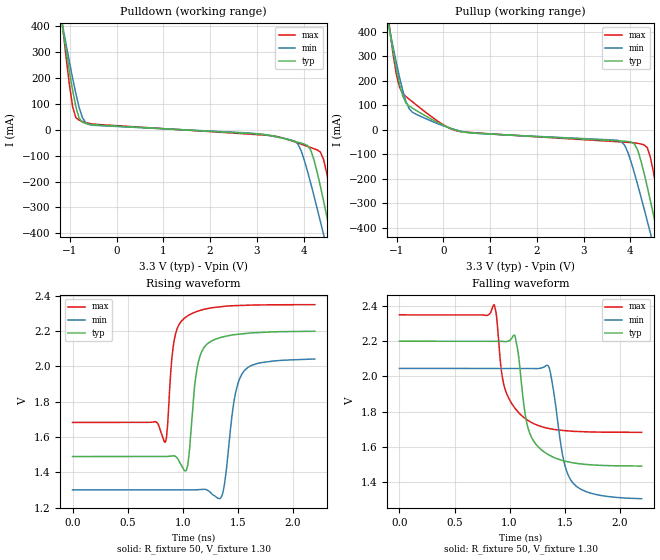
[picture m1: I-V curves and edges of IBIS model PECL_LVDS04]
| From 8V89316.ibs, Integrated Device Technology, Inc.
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[Model]   PECL_LVDS04
|LVPECL Driver
Model_type   Output_ECL
Polarity   Non-Inverting
|   typ   min   max
C_comp   2pF   1.5pF   2.5pF
Vmeas = 1.95V
Rref = 50
Cref = 0
Vref = 1.3V
|   typ   min   max
[Voltage range]   3.3V   3.135V   3.465V
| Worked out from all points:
|   rising waveform, R_fixture 50, V_fixture 1.30: 20-80 % time 82.3ps typ, 95.1ps min, 74.8ps max; typ from 1.49 V to 2.2 V
|   falling waveform, R_fixture 50, V_fixture 1.30: 20-80 % time 127ps typ, 118ps min, 154ps max; typ from 2.2 V to 1.49 V
[Pulldown]
|Voltage   I (typ)   I (min)   I (max)
-3.3V     3.045A     2.601A     4.065A
-1.146V   383.9mA    395mA      387.6mA
-939.2mV  152.8mA    199.5mA    89.52mA
-801.5mV  45.92mA    87.39mA    37.53mA
-594.9mV  22.04mA    20.74mA    25.14mA
3.811V    -44.66mA   -43.56mA   -46.44mA
3.949V    -51.54mA   -81mA      -55.19mA
4.156V    -79.05mA   -207.7mA   -68.56mA
4.431V    -276.5mA   -406.1mA   -115.7mA
4.51V     -344.5mA   -464.8mA   -180.2mA
4.928V    -719.3mA   -781.2mA   -653.8mA
6.6V      -2.246A    -2.062A    -2.647A
[Pullup]
|Voltage   I (typ)   I (min)   I (max)
-3.3V     3.045A     2.599A     4.069A
-1.215V   477.4mA    471.2mA    517.2mA
-1.146V   397.5mA    404.2mA    408.4mA
-939.2mV  186.3mA    215mA      174.1mA
-732.6mV  97.14mA    85.96mA    125.1mA
231.3mV   319.2uA    1.841mA    -1.041mA
3.811V    -45.71mA   -48.83mA   -49.45mA
4.156V    -82.37mA   -223.7mA   -54.98mA
4.431V    -291.9mA   -423.4mA   -114.3mA
4.51V     -360.5mA   -482.3mA   -189.3mA
4.928V    -736.5mA   -799.2mA   -669.8mA
6.6V      -2.267A    -2.086A    -2.663A
[Ramp]
|   typ   min   max
dV/dt_r   0.633/1.219n   0.632/0.165n   0.623/1.126n
dV/dt_f   0.597/0.256n   0.609/0.216n   0.582/0.272n
R_load =   50.0000
[Rising Waveform]
R_fixture = 50
V_fixture = 1.30   | VCC_typ - 2V
V_fixture_max = 1.465   | VCC_max - 2V
V_fixture_min = 1.135   | VCC_min - 2V
C_fixture = 0.0p
| Time   typ   min   max
0s        1.489V     1.3V       1.682V
753ps     1.489V     1.3V       1.687V
841ps     1.489V     1.3V       1.571V
924ps     1.493V     1.3V       2.153V
1.028ns   1.408V     1.3V       2.279V
1.142ns   2.024V     1.301V     2.314V
1.341ns   2.163V     1.252V     2.338V
1.468ns   2.179V     1.811V     2.344V
1.545ns   2.185V     1.963V     2.346V
2.199ns   2.199V     2.042V     2.349V
[Falling Waveform]
R_fixture = 50
V_fixture = 1.30   | VCC_typ - 2V
V_fixture_max = 1.465   | VCC_max - 2V
V_fixture_min = 1.135   | VCC_min - 2V
C_fixture = 0.0p
| Time   typ   min   max
0s        2.201V     2.046V     2.352V
861ps     2.201V     2.046V     2.409V
935ps     2.2V       2.046V     1.991V
1.046ns   2.234V     2.046V     1.822V
1.164ns   1.714V     2.046V     1.75V
1.345ns   1.556V     2.063V     1.705V
1.385ns   1.543V     1.973V     1.7V
1.49ns    1.519V     1.524V     1.691V
1.567ns   1.508V     1.399V     1.687V
2.199ns   1.489V     1.302V     1.681V
